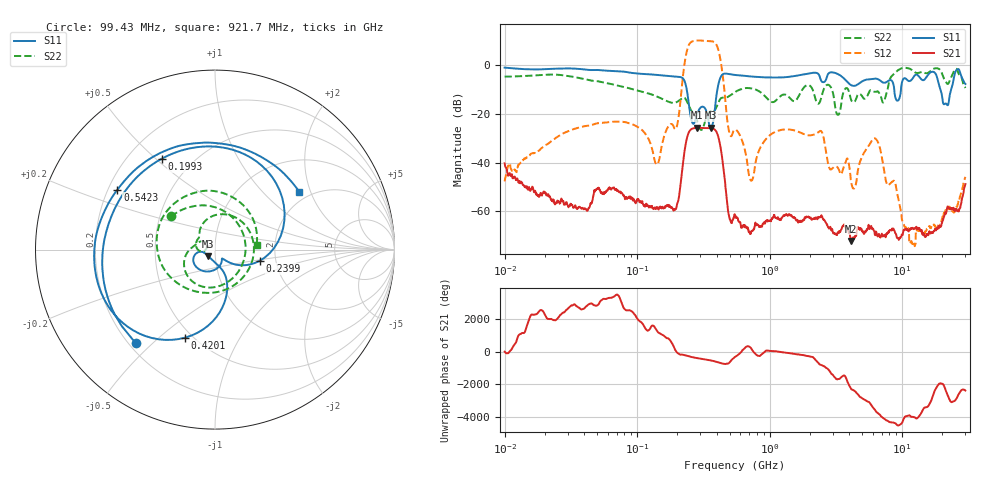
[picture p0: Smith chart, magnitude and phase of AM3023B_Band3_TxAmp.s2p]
# Hz S DB R 50.0
!freq dBS11 angS11 dBS21 angS21 dBS12 angS12 dBS22 angS22
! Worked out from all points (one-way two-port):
!   1601 points, 10 MHz to 30 GHz, reference 50 ohm
!   highest |S21| = -25.61 dB at 282.9 MHz (marker M1); lowest = -72.1 dB at 4.094 GHz (marker M2)
!   lowest |S11| = -25.6 dB at 359.8 MHz (marker M3), VSWR 1.11, Z = 46.3 - j3.46 ohm
!   |S11| at or under -10 dB: 236.9 MHz to 402.9 MHz (166 MHz wide, 51.9 % of centre); 8.72 GHz to 9.791 GHz (1.071 GHz wide, 11.6 % of centre); 19.49 GHz to 23.4 GHz (3.913 GHz wide, 18.2 % of centre)
!   |S22| runs from -26.5 to -0.9 dB; largest |S21 - S12| = 3.3
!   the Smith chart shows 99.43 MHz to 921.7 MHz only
!   S11 on the Smith chart (normalised r, x): 99.43 MHz: 0.23, -0.44; 199.3 MHz: 0.34, +0.52; 239.9 MHz: 1.65, -0.22; 420.1 MHz: 0.46, -0.61; 542.3 MHz: 0.24, +0.27; 921.7 MHz: 1.75, +1.67
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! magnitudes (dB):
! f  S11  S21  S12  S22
! 10 MHz  -0.9  -40.2  -47.7  -4.6
! 38.04 MHz  -1.5  -58.9  -25.3  -5.4
! 99.43 MHz  -3.3  -55.9  -25.1  -10.2
! 144.7 MHz  -4.0  -59.1  -39.9  -13.0
! 199.3 MHz  -4.6  -57.6  -25.0  -15.0
! 239.9 MHz  -11.8  -29.0  6.9  -15.3
! 282.9 MHz  -20.1  -25.6  10.3  -22.5
! 359.8 MHz  -25.6  -25.8  10.0  -19.0
! 420.1 MHz  -5.7  -31.9  3.9  -14.1
! 490.6 MHz  -3.5  -61.0  -26.4  -12.7
! 542.3 MHz  -3.9  -61.2  -26.5  -11.1
! 547.7 MHz  -3.9  -61.5  -26.4  -11.0
! 724.9 MHz  -4.6  -68.2  -47.4  -9.4
! 921.7 MHz  -4.9  -65.0  -30.8  -12.6
! 2.084 GHz  -3.1  -63.3  -28.7  -9.3
! 4.094 GHz  -8.0  -72.1  -46.9  -13.7
! 6.202 GHz  -5.4  -69.1  -30.0  -10.9
! 7.926 GHz  -6.2  -68.1  -49.1  -7.1
! 12.13 GHz  -5.0  -67.1  -72.4  -2.3
! 17.39 GHz  -2.7  -68.1  -65.7  -1.3
! 21.35 GHz  -15.6  -61.0  -59.5  -6.8
! 30 GHz  -7.6  -48.8  -45.8  -9.3
